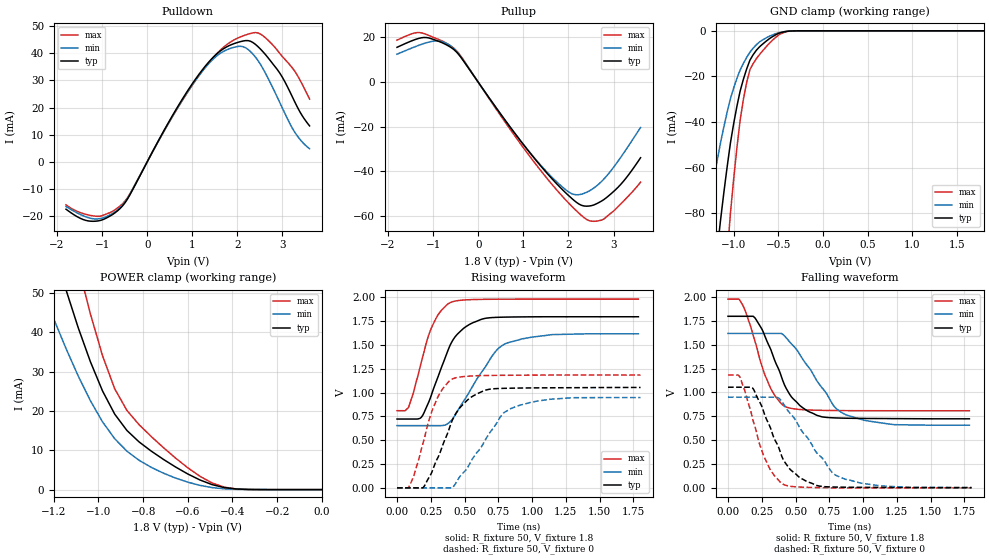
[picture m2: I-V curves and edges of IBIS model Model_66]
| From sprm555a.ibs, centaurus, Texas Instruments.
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| Model based on original model for BCSHTLTCSCDVPBFZ_SSGFV
|   Sub model SR10_11MA_10PER_1P8
[model]   Model_66
|[Description]  [1.8V-3-STATE-X-SLOW:11MA, IND, 10%]
|   Slow slew rate (SR[1:0] = "01"), 0.73 * RExt = 1.325 * Iout
|   (I[2:0] = "110"), 11mA nominal with Rext = 50R, ,Industrial
|   temperature range (-40C to 125C, 25C nominal),10% power supply
|   tolerance
|[Input Load]
|[Output Drive] SLOW:11MA
|Voltage   1.8V
|Mode   3-STATE
Model_type   3-state
Polarity   Non-Inverting
Enable   Active-Low
Cref =  15pF
Rref =  100.0000M
Vref =  0V
Vmeas =  0.9
C_comp   1.851324p   1.663768p   1.973575p
[Temperature Range]   25   125   -40
[Voltage Range]   1.8   1.62   1.98
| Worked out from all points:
|   slope of the pulldown table from 0 to 0.27 V, typ, clamps not added: 32 ohm
|   slope of the pullup table from 0 to 0.27 V, typ, clamps not added: 34.5 ohm
|   GND clamp passes 1 mA (typ) near -0.49 V on its own axis
|   POWER clamp passes 1 mA (typ) near -0.47 V on its own axis
|   rising waveform, R_fixture 50, V_fixture 1.8: 20-80 % time 183ps typ, 260ps min, 148ps max; typ from 0.722 V to 1.79 V
|   rising waveform, R_fixture 50, V_fixture 0: 20-80 % time 197ps typ, 261ps min, 153ps max; typ from 0 V to 1.05 V
|   falling waveform, R_fixture 50, V_fixture 1.8: 20-80 % time 204ps typ, 270ps min, 161ps max; typ from 1.8 V to 0.724 V
|   falling waveform, R_fixture 50, V_fixture 0: 20-80 % time 197ps typ, 282ps min, 158ps max; typ from 1.05 V to 0.002 V
[POWER_clamp]
-1.8V     194.9mA    137.1mA    262.8mA
-1.236V   68.49mA    48.51mA    92.67mA
-1.145V   50.76mA    35.86mA    69.65mA
-1.127V   47.56mA    33.54mA    65.34mA
-1.055V   35.4mA     24.69mA    48.69mA
-981.8mV  25.06mA    17.2mA     34.01mA
-927.3mV  19.17mA    12.93mA    25.61mA
-872.7mV  15.03mA    9.767mA    20.12mA
-818.2mV  12.12mA    7.45mA     16.5mA
-654.5mV  5.738mA    2.93mA     8.003mA
-436.4mV  508.2uA    199.4uA    613uA
0V        2.273nA    15.95nA    16.67nA
[Pulldown]
-1.8V     -17.41mA   -16.43mA   -15.81mA
-1.145V   -21.83mA   -21.01mA   -19.99mA
-545.5mV  -16.18mA   -15.87mA   -15.39mA
545.5mV   16.61mA    16.34mA    16.22mA
1.091V    30.91mA    30.47mA    30.41mA
1.527V    39.51mA    38.78mA    39.54mA
1.964V    43.74mA    42.34mA    45.21mA
2.291V    44.39mA    40.59mA    47.27mA
2.618V    39.56mA    32.74mA    45.71mA
2.945V    32.54mA    21.66mA    39.78mA
3.218V    23.95mA    12.39mA    34.58mA
3.6V      13.24mA    4.837mA    23.12mA
[Pullup]
-1.8V     15.59mA    12.51mA    18.8mA
-1.309V   19.63mA    16.55mA    22.2mA
-927.3mV  18.65mA    18.46mA    19.52mA
-600mV    15.48mA    16.08mA    16.11mA
-381.8mV  11.09mA    11.19mA    11.57mA
1.2V      -32.98mA   -32.79mA   -34.72mA
1.745V    -45.62mA   -44.74mA   -48.37mA
2.127V    -52.98mA   -50.3mA    -56.63mA
2.455V    -55.48mA   -48.79mA   -61.96mA
2.727V    -53.34mA   -44.61mA   -61.81mA
3.164V    -45.71mA   -33.58mA   -54.45mA
3.6V      -33.84mA   -20.34mA   -44.81mA
[GND_clamp]
-1.8V     -346.1mA   -209.3mA   -568.3mA
-1.327V   -149.7mA   -89.03mA   -250.9mA
-1.291V   -135.6mA   -80.47mA   -227.5mA
-1.145V   -82.35mA   -48.67mA   -137.7mA
-1.073V   -59.44mA   -35.55mA   -97.96mA
-1.036V   -49.1mA    -29.72mA   -79.9mA
-927.3mV  -26.31mA   -17.11mA   -38.99mA
-854.5mV  -16.67mA   -11.64mA   -22.56mA
-818.2mV  -12.86mA   -9.351mA   -16.98mA
-672.7mV  -5.705mA   -3.913mA   -8.624mA
-381.8mV  -120.4uA   -129uA     -167.4uA
1.8V      2.273nA    454nA      6.646nA
[Ramp]
dV/dt_f 0.64902262/0.20511691n 0.58247743/0.27170642n 0.70409001/0.16183392n
dV/dt_r  0.6356503/0.19802127n 0.57368439/0.2640321n 0.71173477/0.15342535n
R_load = 50
[Rising Waveform]
R_fixture = 50
V_fixture = 1.8
V_fixture_min = 1.62
V_fixture_max = 1.98
0s        722mV      652.9mV    809.4mV
85ps      722mV      652.9mV    842.6mV
180.5ps   741.3mV    652.9mV    1.324V
286.6ps   1.101V     652.9mV    1.772V
398.4ps   1.512V     700.8mV    1.946V
559.8ps   1.731V     1.065V     1.975V
727.6ps   1.788V     1.428V     1.979V
804.4ps   1.791V     1.514V     1.979V
1.147ns   1.795V     1.608V     1.98V
1.787ns   1.795V     1.616V     1.98V
[Rising Waveform]
R_fixture = 50
V_fixture = 0
V_fixture_min = 0
V_fixture_max = 0
0s        0V         0V         0V
96ps      0V         0V         29.85mV
200.9ps   15.9mV     0V         509.4mV
304.3ps   322.4mV    0V         959.5mV
415.2ps   728mV      9.674mV    1.145V
587.9ps   983.2mV    364.5mV    1.176V
776.1ps   1.044V     765.8mV    1.181V
841.8ps   1.046V     831.3mV    1.181V
1.131ns   1.05V      929mV      1.183V
1.803ns   1.053V     947.3mV    1.184V
[Falling Waveform]
R_fixture = 50
V_fixture = 1.8
V_fixture_min = 1.62
V_fixture_max = 1.98
0s        1.799V     1.619V     1.979V
81.9ps    1.799V     1.619V     1.979V
200.3ps   1.781V     1.619V     1.533V
314.9ps   1.456V     1.619V     1.046V
429.7ps   1.046V     1.575V     848.5mV
605.3ps   794.7mV    1.25V      815.9mV
783.5ps   734.2mV    858.2mV    810.9mV
877ps     730.3mV    763.9mV    809.8mV
1.231ns   726.2mV    662.6mV    808.6mV
1.787ns   724.1mV    657.3mV    808.4mV
[Falling Waveform]
R_fixture = 50
V_fixture = 0
V_fixture_min = 0
V_fixture_max = 0
0s        1.055V     951.4mV    1.183V
88.6ps    1.055V     951.4mV    1.161V
187.3ps   1.037V     951.4mV    696.8mV
235.6ps   897.8mV    951.4mV    450.4mV
297.3ps   683.6mV    951.4mV    235mV
410.1ps   293.3mV    880.8mV    36.4mV
575.6ps   72.59mV    545.8mV    5.858mV
801ps     8.164mV    129.9mV    0V
1.153ns   4.468mV    19.03mV    0V
1.803ns   2.359mV    3.18mV     0V
